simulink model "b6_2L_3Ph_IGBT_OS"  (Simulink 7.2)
settings: Solver=ode3  SolverMode=SingleTasking  StartTime=0.0  StopTime=0.1  FixedStep=10e-6  MaxStep=1e-5  RelTol=1e-4  AbsTol=1e-4
PreLoadFcn:
  | INIT_B6_2L_3Ph_IGBT_OS
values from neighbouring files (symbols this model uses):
  C = 10e-3*1    (= 0.01)    [INIT_B6_2L_3Ph_IGBT_OS.m]    (also in INIT_B6_3L_3Ph_IGBT_OS.m; INIT_MMC_100L.m = 0.005; INIT_MMC_200L.m = 0.005; INIT_MMC_20L.m)
  FS = 900    [INIT_B6_2L_3Ph_IGBT_OS.m]    (also in INIT_B6_3L_3Ph_IGBT_OS.m; INIT_PWM_2L.m = 1000; INIT_PWM_3L.m = 1000; INIT_PWM_Con.m = 1000)
  I_B = INS    [INIT_B6_2L_3Ph_IGBT_OS.m]    (also in INIT_B6_3L_3Ph_IGBT_OS.m; INIT_PWM_2L.m = INP; INIT_PWM_3L.m = INP; INIT_PWM_Con.m = INP)
  IDC = PDC/VDC    (= 166.666666667)    [INIT_B6_2L_3Ph_IGBT_OS.m]    (also in INIT_B6_3L_3Ph_IGBT_OS.m = 100; INIT_PWM_2L.m = 16.6666666667; INIT_PWM_3L.m = 83.3333333333; INIT_PWM_Con.m = 83.3333333333)
  LS = 1e-3    (= 0.001)    [INIT_B6_2L_3Ph_IGBT_OS.m]    (also in INIT_B6_3L_3Ph_IGBT_OS.m; INIT_MMC_100L.m = 0.025; INIT_MMC_200L.m = 0.025; INIT_MMC_20L.m = 0.0025)
  UC0 = 600    [INIT_B6_2L_3Ph_IGBT_OS.m]    (also in INIT_B6_3L_3Ph_IGBT_OS.m = 500; INIT_MMC_100L.m = 6800; INIT_MMC_200L.m = 3400; INIT_MMC_20L.m = 5000)
  UNS = ULLP/sqrt(3)    [INIT_B6_2L_3Ph_IGBT_OS.m]    (also in INIT_B6_3L_3Ph_IGBT_OS.m; INIT_MMC_100L.m = ULLP/sqrt(3)*340/400; INIT_MMC_200L.m = ULLP/sqrt(3)*340/400; INIT_MMC_20L.m)

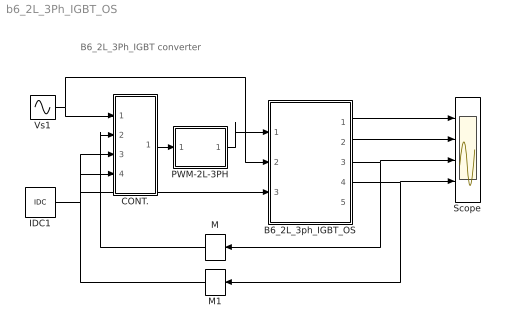
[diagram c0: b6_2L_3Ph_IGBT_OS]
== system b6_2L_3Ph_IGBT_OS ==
  note: B6_2L_3Ph_IGBT converter
  B6_2L_3ph_IGBT_OS : Subsystem  mask(B6 2-Level IGBT 3-Phase Converter){LS=LS, C=C, UC0=UC0, RL=1e6}
      mask prompts: LS "Source Inductance"; C "Load Cap"; UC0 "Initial Cap Voltage"; RL "Load Resistance"
      mask help: Input Vector u: u[0]= IGBT1.gate u[1]= IGBT2.gate u[2]= IGBT3.gate u[3]= IGBT4.gate u[4]= IGBT5.gate u[5]= IGBT6.gate u[6]= V1.V u[7]= V2.V u[8]= V3.V u[9]= IDC.i Output Vector y: y[0]= T1.I y[1]= D1.I y[2]= T1.V y[3]= T2.I y[4]= D2.I y[5]= T2.V y[6]= LS1.I y[7]= LS2.I y[8]= LS3.I y[9]= DC.V y[10]= Va.V y[11]= Vb.V y[12]= Vc.V Parameter Vector p: p[0]= Ls.L p[1]= C1.C p[2]= C1.vC0 p[3]= R1.r You can pause the simulation during running, change the Parameters you want and continue the Simulation
  CONT. : Subsystem
  IDC1 : Constant  Value=IDC
  M : Memory  Orientation=left
  M1 : Memory  Orientation=left
  PWM-2L-3PH : Subsystem  mask(PWM3-2L-3PH){FT=FS, PHT=0, DT=1e-6}
      mask prompts: FT "Triangular Frequency"; PHT "Trian. Phase Angle (Degree)"; DT "Dead Time"
      mask help: Pulse Width Modulation for 3 Phase Converter
  Scope : Scope  NumInputPorts=4
  Vs1 : Sin  Amplitude=UNS  Frequency=50*2*pi  Phase="[0  -2*pi/3   -4*pi/3]"  SampleTime=0
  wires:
  Vs1/1 -> CONT./1(UN), B6_2L_3ph_IGBT_OS/2(vS)
  IDC1/1 -> CONT./4(Id*), B6_2L_3ph_IGBT_OS/3(iDC)
  CONT./1(A) -> PWM-2L-3PH/1(In4)
  PWM-2L-3PH/1(Out1) -> B6_2L_3ph_IGBT_OS/1(SWs)
  B6_2L_3ph_IGBT_OS/3(iLs) -> Scope/3, M/1
  M/1 -> CONT./2(Iwr)
  B6_2L_3ph_IGBT_OS/1(iT1,iD1,vT1) -> Scope/1
  B6_2L_3ph_IGBT_OS/2(iT2,iD2,vT2) -> Scope/2
  B6_2L_3ph_IGBT_OS/4(vDC) -> Scope/4, M1/1
  M1/1 -> CONT./3(UDC)

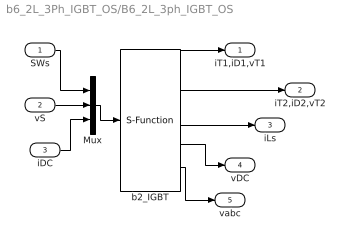
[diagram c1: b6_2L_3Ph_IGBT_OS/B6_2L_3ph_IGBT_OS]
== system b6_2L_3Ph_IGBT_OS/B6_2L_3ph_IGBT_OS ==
  SWs : Inport  OutDataType=sfix(16)  OutScaling=2^0
  vS : Inport  Port=2  OutDataType=sfix(16)  OutScaling=2^0
  iDC : Inport  Port=3  OutDataType=sfix(16)  OutScaling=2^0
  Mux : Mux  Inputs="[6  3  1]"
  b2_IGBT : S-Function  FunctionName=s_b6_2L_3Ph_IGBT_OS  Parameters="[ LS  C  UC0 RL]"  EnableBusSupport=off
  iT1,iD1,vT1 : Outport  OutDataType=sfix(16)  OutScaling=2^0
  iT2,iD2,vT2 : Outport  Port=2  OutDataType=sfix(16)  OutScaling=2^0
  iLs : Outport  Port=3  OutDataType=sfix(16)  OutScaling=2^0
  vDC : Outport  Port=4  OutDataType=sfix(16)  OutScaling=2^0
  vabc : Outport  Port=5  OutDataType=sfix(16)  OutScaling=2^0
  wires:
  b2_IGBT/5 -> vabc/1
  SWs/1 -> Mux/1
  vS/1 -> Mux/2
  b2_IGBT/1 -> iT1,iD1,vT1/1
  b2_IGBT/2 -> iT2,iD2,vT2/1
  b2_IGBT/3 -> iLs/1
  iDC/1 -> Mux/3
  Mux/1 -> b2_IGBT/1
  b2_IGBT/4 -> vDC/1

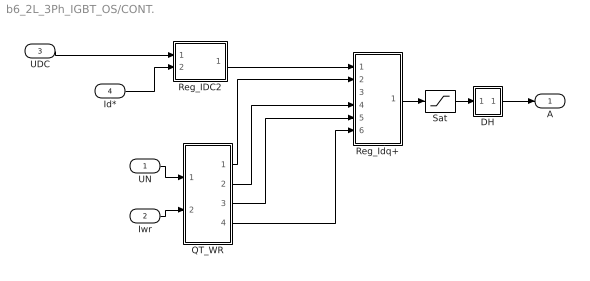
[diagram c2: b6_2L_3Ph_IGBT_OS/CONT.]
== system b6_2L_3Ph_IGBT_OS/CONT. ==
  UN : Inport
  Iwr : Inport  Port=2
  UDC : Inport  Port=3
  Id* : Inport  Port=4
  DH : Subsystem
  QT_WR : Subsystem
  Reg_IDC2 : Subsystem
  Reg_Idq+ : Subsystem
  Sat : Saturate  UpperLimit=1.5  LowerLimit=-1.5
  A : Outport
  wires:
  Sat/1 -> DH/1(I)
  Reg_Idq+/1(A+) -> Sat/1
  Id*/1 -> Reg_IDC2/2(Id*)
  DH/1(O) -> A/1
  UDC/1 -> Reg_IDC2/1(UDC)
  UN/1 -> QT_WR/1(UN)
  Iwr/1 -> QT_WR/2(I_WR)
  Reg_IDC2/1(Id1*) -> Reg_Idq+/1(Id1*)
  QT_WR/3(th1) -> Reg_Idq+/5(th)
  QT_WR/2(Iq1) -> Reg_Idq+/4(Iq1)
  QT_WR/1(Id1) -> Reg_Idq+/2(Id1)
  QT_WR/4(Ud) -> Reg_Idq+/6(Ud)

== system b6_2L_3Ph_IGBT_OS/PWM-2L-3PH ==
  In4 : Inport  OutDataType=sfix(16)  OutScaling=2^0
  Demux : Demux  Outputs=3
  Mux : Mux  Inputs=3
  PWM-2L-1PH : Subsystem  mask(PWM-2L-1PH){FT=FT, PHT=PHT, DT=DT}
      mask prompts: FT "Triangular Frequency"; PHT "Trian. Phase Angle (Degree)"; DT "Dead Time"
      mask help: Pulse Width Modulation for 1 Phase Converter
  PWM-2L-1PH1 : Subsystem  mask(PWM-2L-1PH){FT=FT, PHT=PHT, DT=DT}
      mask prompts: FT "Triangular Frequency"; PHT "Trian. Phase Angle (Degree)"; DT "Dead Time"
      mask help: Pulse Width Modulation for 1 Phase Converter
  PWM-2L-1PH2 : Subsystem  mask(PWM-2L-1PH){FT=FT, PHT=PHT, DT=DT}
      mask prompts: FT "Triangular Frequency"; PHT "Trian. Phase Angle (Degree)"; DT "Dead Time"
      mask help: Pulse Width Modulation for 1 Phase Converter
  Out1 : Outport
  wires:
  In4/1 -> Demux/1
  Demux/3 -> PWM-2L-1PH2/1(In1)
  Demux/2 -> PWM-2L-1PH1/1(In1)
  Demux/1 -> PWM-2L-1PH/1(In1)
  PWM-2L-1PH1/1(Out1) -> Mux/2
  PWM-2L-1PH/1(Out1) -> Mux/1
  PWM-2L-1PH2/1(Out1) -> Mux/3
  Mux/1 -> Out1/1

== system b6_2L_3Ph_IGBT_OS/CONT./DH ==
  I : Inport
  Gain : Gain  Gain=0.5
  MinMax : MinMax
  MinMax1 : MinMax  Function=max
  Sum6 : Sum  Inputs=--
  Sum7 : Sum
  O : Outport  InitialOutput=0
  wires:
  I/1 -> MinMax1/1, MinMax/1, Sum7/1
  MinMax/1 -> Sum6/1
  MinMax1/1 -> Sum6/2
  Sum6/1 -> Gain/1
  Gain/1 -> Sum7/2
  Sum7/1 -> O/1

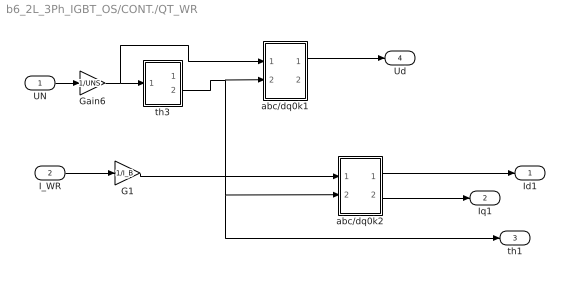
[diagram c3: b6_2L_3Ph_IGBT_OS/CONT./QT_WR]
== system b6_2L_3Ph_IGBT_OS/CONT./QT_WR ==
  UN : Inport
  I_WR : Inport  Port=2
  G1 : Gain  Gain=1/I_B
  Gain6 : Gain  Gain=1/UNS
  abc/dq0k1 : Subsystem
  abc/dq0k2 : Subsystem
  th3 : Subsystem
  Id1 : Outport
  Iq1 : Outport  Port=2
  th1 : Outport  Port=3
  Ud : Outport  Port=4
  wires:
  th3/2(th) -> abc/dq0k2/2(th), th1/1, abc/dq0k1/2(th)
  I_WR/1 -> G1/1
  G1/1 -> abc/dq0k2/1(a)
  UN/1 -> Gain6/1
  Gain6/1 -> th3/1(abc), abc/dq0k1/1(a)
  abc/dq0k2/1(dk) -> Id1/1
  abc/dq0k2/2(qk) -> Iq1/1
  abc/dq0k1/1(dk) -> Ud/1

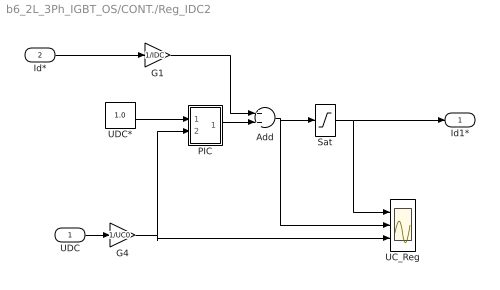
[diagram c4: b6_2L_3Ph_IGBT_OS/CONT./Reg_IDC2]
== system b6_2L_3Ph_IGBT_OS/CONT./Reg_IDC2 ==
  UDC : Inport
  Id* : Inport  Port=2
  Add : Sum
  G1 : Gain  Gain=1/IDC
  G4 : Gain  Gain=1/UC0
  PIC : Subsystem  mask(PI-controller){Kp=1, Ki=10, lim=2, Ts=-1}
      mask prompts: Kp "Proportional gain (Kp)"; Ki "Integral gain (Ki)"; lim "Output limit"; Ts "Sampling time (s)"
      mask help: Proportional-Integral Controller
  Sat : Saturate  UpperLimit=2  LowerLimit=-2
  UC_Reg : Scope  NumInputPorts=3
  UDC* : Constant  Value=1.0
  Id1* : Outport
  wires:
  Id*/1 -> G1/1
  PIC/1(e*) -> Add/2
  Sat/1 -> Id1*/1, UC_Reg/1
  Add/1 -> Sat/1, UC_Reg/2
  G4/1 -> UC_Reg/3, PIC/2(c)
  UDC*/1 -> PIC/1(c*)
  UDC/1 -> G4/1
  G1/1 -> Add/1

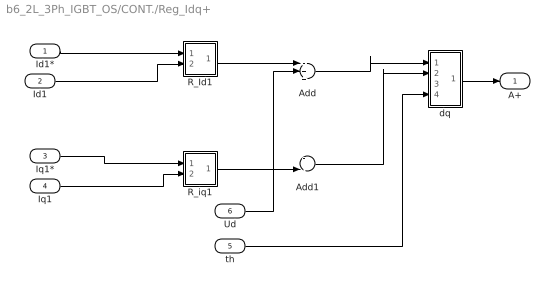
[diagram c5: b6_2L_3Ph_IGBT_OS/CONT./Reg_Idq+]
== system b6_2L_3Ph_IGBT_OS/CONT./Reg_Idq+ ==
  Id1* : Inport
  Id1 : Inport  Port=2
  Iq1* : Inport  Port=3
  Iq1 : Inport  Port=4
  th : Inport  Port=5
  Ud : Inport  Port=6
  Add : Sum  Inputs=-++
  Add1 : Sum  Inputs=--
  R_Id1 : Subsystem  mask(PI-controller){Kp=0.1, Ki=200, lim=2, Ts=-1}
      mask prompts: Kp "Proportional gain (Kp)"; Ki "Integral gain (Ki)"; lim "Output limit"; Ts "Sampling time (s)"
      mask help: Proportional-Integral Controller
  R_iq1 : Subsystem  mask(PI-controller){Kp=0.1, Ki=200, lim=2, Ts=-2}
      mask prompts: Kp "Proportional gain (Kp)"; Ki "Integral gain (Ki)"; lim "Output limit"; Ts "Sampling time (s)"
      mask help: Proportional-Integral Controller
  dq : Subsystem
  A+ : Outport
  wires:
  Iq1/1 -> R_iq1/2(c)
  Iq1*/1 -> R_iq1/1(c*)
  Id1/1 -> R_Id1/2(c)
  Id1*/1 -> R_Id1/1(c*)
  dq/1(a) -> A+/1
  th/1 -> dq/4(th)
  R_Id1/1(e*) -> Add/1
  R_iq1/1(e*) -> Add1/2
  Add/1 -> dq/1(dk)
  Add1/1 -> dq/2(qk)
  Ud/1 -> Add/2

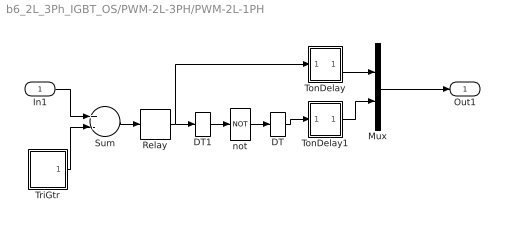
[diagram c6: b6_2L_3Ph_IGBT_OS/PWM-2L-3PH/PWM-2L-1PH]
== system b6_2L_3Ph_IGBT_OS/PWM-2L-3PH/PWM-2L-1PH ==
  In1 : Inport  OutDataType=sfix(16)  OutScaling=2^0
  DT : DataTypeConversion
  DT1 : DataTypeConversion
  Mux : Mux  Inputs=2
  Relay : Relay  OutDataType=sfix(16)  OutScaling=2^0
  Sum : Sum  Inputs=+-  OutDataType=sfix(16)  OutScaling=2^0
  TonDelay : Subsystem  mask(TonDelay){DT=DT}
      mask prompts: DT "Dead Time"
      mask help: Turn on dead time to protect against short circuit of the converter leg
  TonDelay1 : Subsystem  mask(TonDelay){DT=DT}
      mask prompts: DT "Dead Time"
      mask help: Turn on dead time to protect against short circuit of the converter leg
  TriGtr : Subsystem  mask(TriGtr){T=1/FT, Td=PHT/FT/360}
      mask prompts: T "Period Time"; Td "Time Delay"
      mask help: Triangular Wave Generator with variable time delay
  not : Logic  Operator=NOT  Inputs=1
  Out1 : Outport  InitialOutput=0
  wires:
  Mux/1 -> Out1/1
  TonDelay/1(s1d) -> Mux/1
  Relay/1 -> TonDelay/1(s1), DT1/1
  TonDelay1/1(s1d) -> Mux/2
  not/1 -> DT/1
  Sum/1 -> Relay/1
  TriGtr/1(O) -> Sum/2
  In1/1 -> Sum/1
  DT/1 -> TonDelay1/1(s1)
  DT1/1 -> not/1

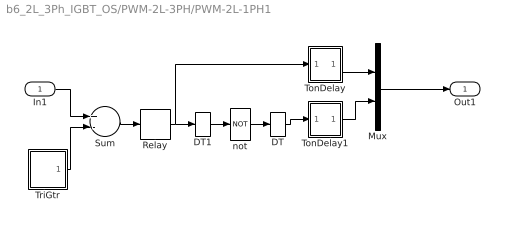
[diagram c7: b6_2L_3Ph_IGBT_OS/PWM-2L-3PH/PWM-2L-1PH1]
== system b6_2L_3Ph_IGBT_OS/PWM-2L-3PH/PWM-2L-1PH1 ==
  In1 : Inport  OutDataType=sfix(16)  OutScaling=2^0
  DT : DataTypeConversion
  DT1 : DataTypeConversion
  Mux : Mux  Inputs=2
  Relay : Relay  OutDataType=sfix(16)  OutScaling=2^0
  Sum : Sum  Inputs=+-  OutDataType=sfix(16)  OutScaling=2^0
  TonDelay : Subsystem  mask(TonDelay){DT=DT}
      mask prompts: DT "Dead Time"
      mask help: Turn on dead time to protect against short circuit of the converter leg
  TonDelay1 : Subsystem  mask(TonDelay){DT=DT}
      mask prompts: DT "Dead Time"
      mask help: Turn on dead time to protect against short circuit of the converter leg
  TriGtr : Subsystem  mask(TriGtr){T=1/FT, Td=PHT/FT/360}
      mask prompts: T "Period Time"; Td "Time Delay"
      mask help: Triangular Wave Generator with variable time delay
  not : Logic  Operator=NOT  Inputs=1
  Out1 : Outport  InitialOutput=0
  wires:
  DT1/1 -> not/1
  DT/1 -> TonDelay1/1(s1)
  In1/1 -> Sum/1
  TriGtr/1(O) -> Sum/2
  Sum/1 -> Relay/1
  not/1 -> DT/1
  TonDelay1/1(s1d) -> Mux/2
  Relay/1 -> DT1/1, TonDelay/1(s1)
  TonDelay/1(s1d) -> Mux/1
  Mux/1 -> Out1/1

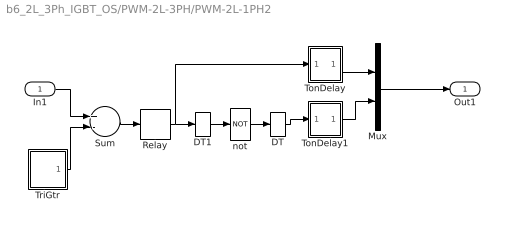
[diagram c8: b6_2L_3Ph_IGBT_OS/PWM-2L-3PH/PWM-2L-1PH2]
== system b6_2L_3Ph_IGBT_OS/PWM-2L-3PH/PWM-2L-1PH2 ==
  In1 : Inport  OutDataType=sfix(16)  OutScaling=2^0
  DT : DataTypeConversion
  DT1 : DataTypeConversion
  Mux : Mux  Inputs=2
  Relay : Relay  OutDataType=sfix(16)  OutScaling=2^0
  Sum : Sum  Inputs=+-  OutDataType=sfix(16)  OutScaling=2^0
  TonDelay : Subsystem  mask(TonDelay){DT=DT}
      mask prompts: DT "Dead Time"
      mask help: Turn on dead time to protect against short circuit of the converter leg
  TonDelay1 : Subsystem  mask(TonDelay){DT=DT}
      mask prompts: DT "Dead Time"
      mask help: Turn on dead time to protect against short circuit of the converter leg
  TriGtr : Subsystem  mask(TriGtr){T=1/FT, Td=PHT/FT/360}
      mask prompts: T "Period Time"; Td "Time Delay"
      mask help: Triangular Wave Generator with variable time delay
  not : Logic  Operator=NOT  Inputs=1
  Out1 : Outport  InitialOutput=0
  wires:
  Mux/1 -> Out1/1
  TonDelay/1(s1d) -> Mux/1
  Relay/1 -> TonDelay/1(s1), DT1/1
  TonDelay1/1(s1d) -> Mux/2
  not/1 -> DT/1
  Sum/1 -> Relay/1
  TriGtr/1(O) -> Sum/2
  In1/1 -> Sum/1
  DT/1 -> TonDelay1/1(s1)
  DT1/1 -> not/1

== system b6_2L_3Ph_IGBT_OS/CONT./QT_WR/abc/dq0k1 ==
  a : Inport
  th : Inport  Port=2
  Demux : Demux  Outputs=3
  Fcn : Fcn  Expr=u(1)*cos(u(3)) + u(2)*sin(u(3))
  Fcn1 : Fcn  Expr=-u(1)*sin(u(3)) + u(2)*cos(u(3))
  K : Gain  Gain="2/3*[1   -.5   -.5;  0   sqrt(3)/2   -sqrt(3)/2;  .5    .5    .5]"  Multiplication=Matrix(K*u)
  Mux1 : Mux  Inputs=3
  dk : Outport
  qk : Outport  Port=2
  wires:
  Demux/2 -> Mux1/2
  Demux/1 -> Mux1/1
  th/1 -> Mux1/3
  Fcn1/1 -> qk/1
  Fcn/1 -> dk/1
  Mux1/1 -> Fcn/1, Fcn1/1
  a/1 -> K/1
  K/1 -> Demux/1

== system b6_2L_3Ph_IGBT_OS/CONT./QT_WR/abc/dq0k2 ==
  a : Inport
  th : Inport  Port=2
  Demux : Demux  Outputs=3
  Fcn : Fcn  Expr=u(1)*cos(u(3)) + u(2)*sin(u(3))
  Fcn1 : Fcn  Expr=-u(1)*sin(u(3)) + u(2)*cos(u(3))
  K : Gain  Gain="2/3*[1   -.5   -.5;  0   sqrt(3)/2   -sqrt(3)/2;  .5    .5    .5]"  Multiplication=Matrix(K*u)
  Mux1 : Mux  Inputs=3
  dk : Outport
  qk : Outport  Port=2
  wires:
  K/1 -> Demux/1
  a/1 -> K/1
  Mux1/1 -> Fcn1/1, Fcn/1
  Fcn/1 -> dk/1
  Fcn1/1 -> qk/1
  th/1 -> Mux1/3
  Demux/1 -> Mux1/1
  Demux/2 -> Mux1/2

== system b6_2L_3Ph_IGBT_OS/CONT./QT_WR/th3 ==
  abc : Inport
  C : ComplexToMagnitudeAngle
  Demux : Demux  Outputs=3
  K : Gain  Gain="2/3*[1   -.5   -.5;  0   sqrt(3)/2   -sqrt(3)/2;  .5    .5    .5]"  Multiplication=Matrix(K*u)
  R : RealImagToComplex
  |u| : Outport
  th : Outport  Port=2
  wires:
  C/2 -> th/1
  R/1 -> C/1
  Demux/2 -> R/2
  Demux/1 -> R/1
  abc/1 -> K/1
  K/1 -> Demux/1
  C/1 -> |u|/1

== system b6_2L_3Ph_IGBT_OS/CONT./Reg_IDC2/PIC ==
  c* : Inport  OutDataType=sfix(16)  OutScaling=2^0
  c : Inport  Port=2  OutDataType=sfix(16)  OutScaling=2^0
  Gain : Gain  Gain=Ki  ParameterDataType=sfix(16)  ParameterScaling=2^0  OutDataType=sfix(16)  OutScaling=2^0
  Gain1 : Gain  Gain=Kp  ParameterDataType=sfix(16)  ParameterScaling=2^0  OutDataType=sfix(16)  OutScaling=2^0
  Integrator : Integrator  UpperSaturationLimit=lim  LowerSaturationLimit=-lim
  Saturation : Saturate  UpperLimit=lim  LowerLimit=-lim
  Sum1 : Sum  Inputs=+-  OutDataType=sfix(16)  OutScaling=2^0
  Sum2 : Sum  OutDataType=sfix(16)  OutScaling=2^0
  e* : Outport  InitialOutput=0
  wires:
  Integrator/1 -> Sum2/2
  c*/1 -> Sum1/1
  c/1 -> Sum1/2
  Saturation/1 -> e*/1
  Sum2/1 -> Saturation/1
  Sum1/1 -> Gain1/1, Gain/1
  Gain1/1 -> Sum2/1
  Gain/1 -> Integrator/1

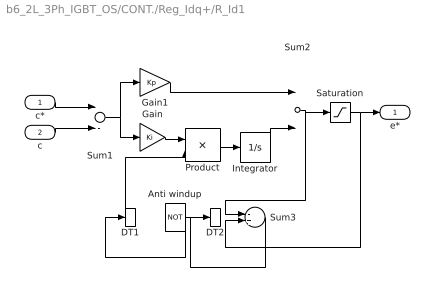
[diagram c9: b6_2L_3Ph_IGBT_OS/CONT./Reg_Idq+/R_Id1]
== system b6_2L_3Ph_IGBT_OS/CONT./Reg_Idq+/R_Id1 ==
  c* : Inport
  c : Inport  Port=2
  Anti windup : Logic  Operator=NOT
  DT1 : DataTypeConversion
  DT2 : DataTypeConversion
  Gain : Gain  Gain=Ki
  Gain1 : Gain  Gain=Kp
  Integrator : Integrator  UpperSaturationLimit=lim  LowerSaturationLimit=-lim
  Product : Product
  Saturation : Saturate  UpperLimit=lim  LowerLimit=-lim
  Sum1 : Sum  Inputs=+-
  Sum2 : Sum
  Sum3 : Sum  Inputs=-+
  e* : Outport  InitialOutput=0
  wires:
  Integrator/1 -> Sum2/2
  c*/1 -> Sum1/1
  c/1 -> Sum1/2
  Saturation/1 -> e*/1, Sum3/2
  Sum2/1 -> Saturation/1, Sum3/1
  Sum1/1 -> Gain1/1, Gain/1
  Gain1/1 -> Sum2/1
  Anti windup/1 -> DT1/1
  DT1/1 -> Product/2
  Gain/1 -> Product/1
  Product/1 -> Integrator/1
  DT2/1 -> Anti windup/1
  Sum3/1 -> DT2/1

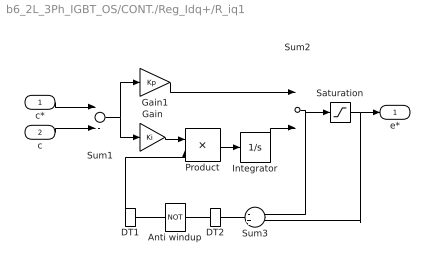
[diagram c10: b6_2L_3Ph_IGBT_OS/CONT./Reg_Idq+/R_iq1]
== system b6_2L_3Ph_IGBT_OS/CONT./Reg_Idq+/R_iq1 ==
  c* : Inport
  c : Inport  Port=2
  Anti windup : Logic  Operator=NOT
  DT1 : DataTypeConversion
  DT2 : DataTypeConversion
  Gain : Gain  Gain=Ki
  Gain1 : Gain  Gain=Kp
  Integrator : Integrator  UpperSaturationLimit=lim  LowerSaturationLimit=-lim
  Product : Product
  Saturation : Saturate  UpperLimit=lim  LowerLimit=-lim
  Sum1 : Sum  Inputs=+-
  Sum2 : Sum
  Sum3 : Sum  Inputs=-+
  e* : Outport  InitialOutput=0
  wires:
  Sum3/1 -> DT2/1
  DT2/1 -> Anti windup/1
  Product/1 -> Integrator/1
  Gain/1 -> Product/1
  DT1/1 -> Product/2
  Anti windup/1 -> DT1/1
  Gain1/1 -> Sum2/1
  Sum1/1 -> Gain/1, Gain1/1
  Sum2/1 -> Sum3/1, Saturation/1
  Saturation/1 -> Sum3/2, e*/1
  c/1 -> Sum1/2
  c*/1 -> Sum1/1
  Integrator/1 -> Sum2/2

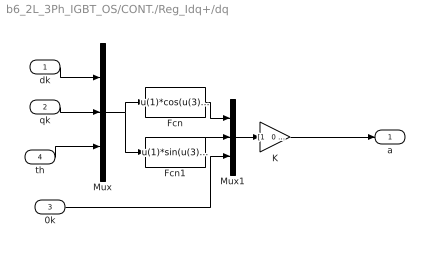
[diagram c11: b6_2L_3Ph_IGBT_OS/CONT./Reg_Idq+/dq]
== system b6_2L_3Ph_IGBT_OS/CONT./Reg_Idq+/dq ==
  dk : Inport
  qk : Inport  Port=2
  0k : Inport  Port=3
  th : Inport  Port=4
  Fcn : Fcn  Expr=u(1)*cos(u(3)) - u(2)*sin(u(3))
  Fcn1 : Fcn  Expr=u(1)*sin(u(3)) + u(2)*cos(u(3))
  K : Gain  Gain="[1   0  1 ;  -.5   sqrt(3)/2    1 ;  -.5    -sqrt(3)/2    1]"  Multiplication=Matrix(K*u)
  Mux : Mux  Inputs=3
  Mux1 : Mux  Inputs=3
  a : Outport
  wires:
  0k/1 -> Mux1/3
  th/1 -> Mux/3
  Fcn1/1 -> Mux1/2
  Fcn/1 -> Mux1/1
  Mux1/1 -> K/1
  K/1 -> a/1
  Mux/1 -> Fcn1/1, Fcn/1
  qk/1 -> Mux/2
  dk/1 -> Mux/1

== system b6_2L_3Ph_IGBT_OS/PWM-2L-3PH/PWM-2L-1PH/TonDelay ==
  s1 : Inport  Orientation=down  OutDataType=sfix(16)  OutScaling=2^0
  Int : Integrator  ExternalReset=falling
  Rel1 : Relay  OnSwitchValue=DT  OutDataType=sfix(16)  OutScaling=2^0
  s1d : Outport  InitialOutput=0
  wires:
  Rel1/1 -> s1d/1
  s1/1 -> Int/1, Int/2
  Int/1 -> Rel1/1

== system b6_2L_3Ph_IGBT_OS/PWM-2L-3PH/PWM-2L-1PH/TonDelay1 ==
  s1 : Inport  Orientation=down  OutDataType=sfix(16)  OutScaling=2^0
  Int : Integrator  ExternalReset=falling
  Rel1 : Relay  OnSwitchValue=DT  OutDataType=sfix(16)  OutScaling=2^0
  s1d : Outport  InitialOutput=0
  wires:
  Rel1/1 -> s1d/1
  s1/1 -> Int/1, Int/2
  Int/1 -> Rel1/1

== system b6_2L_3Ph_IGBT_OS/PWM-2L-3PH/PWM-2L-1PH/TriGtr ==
  Clock : Clock
  S2 : Subsystem
  Sum : Sum  OutDataType=sfix(16)  OutScaling=2^0
  T : Constant  Value=T  OutDataType=sfix(16)  OutScaling=2^0
  Td : Constant  Value=Td  OutDataType=sfix(16)  OutScaling=2^0
  mod : Math  Operator=mod
  O : Outport  InitialOutput=0
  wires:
  Td/1 -> Sum/2
  Sum/1 -> mod/1
  T/1 -> mod/2
  Clock/1 -> Sum/1
  S2/1(O1) -> O/1
  mod/1 -> S2/1(I1)

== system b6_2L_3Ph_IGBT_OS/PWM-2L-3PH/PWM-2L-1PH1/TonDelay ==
  s1 : Inport  Orientation=down  OutDataType=sfix(16)  OutScaling=2^0
  Int : Integrator  ExternalReset=falling
  Rel1 : Relay  OnSwitchValue=DT  OutDataType=sfix(16)  OutScaling=2^0
  s1d : Outport  InitialOutput=0
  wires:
  Int/1 -> Rel1/1
  s1/1 -> Int/2, Int/1
  Rel1/1 -> s1d/1

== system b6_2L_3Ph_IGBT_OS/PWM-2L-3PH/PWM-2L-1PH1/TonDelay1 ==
  s1 : Inport  Orientation=down  OutDataType=sfix(16)  OutScaling=2^0
  Int : Integrator  ExternalReset=falling
  Rel1 : Relay  OnSwitchValue=DT  OutDataType=sfix(16)  OutScaling=2^0
  s1d : Outport  InitialOutput=0
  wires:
  Int/1 -> Rel1/1
  s1/1 -> Int/2, Int/1
  Rel1/1 -> s1d/1

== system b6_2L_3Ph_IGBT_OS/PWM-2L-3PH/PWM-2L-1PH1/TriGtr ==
  Clock : Clock
  S2 : Subsystem
  Sum : Sum  OutDataType=sfix(16)  OutScaling=2^0
  T : Constant  Value=T  OutDataType=sfix(16)  OutScaling=2^0
  Td : Constant  Value=Td  OutDataType=sfix(16)  OutScaling=2^0
  mod : Math  Operator=mod
  O : Outport  InitialOutput=0
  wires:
  mod/1 -> S2/1(I1)
  S2/1(O1) -> O/1
  Clock/1 -> Sum/1
  T/1 -> mod/2
  Sum/1 -> mod/1
  Td/1 -> Sum/2

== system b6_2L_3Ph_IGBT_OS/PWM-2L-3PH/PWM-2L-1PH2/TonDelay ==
  s1 : Inport  Orientation=down  OutDataType=sfix(16)  OutScaling=2^0
  Int : Integrator  ExternalReset=falling
  Rel1 : Relay  OnSwitchValue=DT  OutDataType=sfix(16)  OutScaling=2^0
  s1d : Outport  InitialOutput=0
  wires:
  Rel1/1 -> s1d/1
  s1/1 -> Int/1, Int/2
  Int/1 -> Rel1/1

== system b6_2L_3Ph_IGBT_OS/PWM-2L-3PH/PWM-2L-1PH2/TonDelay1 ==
  s1 : Inport  Orientation=down  OutDataType=sfix(16)  OutScaling=2^0
  Int : Integrator  ExternalReset=falling
  Rel1 : Relay  OnSwitchValue=DT  OutDataType=sfix(16)  OutScaling=2^0
  s1d : Outport  InitialOutput=0
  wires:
  Rel1/1 -> s1d/1
  s1/1 -> Int/1, Int/2
  Int/1 -> Rel1/1

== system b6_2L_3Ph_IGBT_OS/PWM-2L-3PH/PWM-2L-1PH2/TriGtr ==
  Clock : Clock
  S2 : Subsystem
  Sum : Sum  OutDataType=sfix(16)  OutScaling=2^0
  T : Constant  Value=T  OutDataType=sfix(16)  OutScaling=2^0
  Td : Constant  Value=Td  OutDataType=sfix(16)  OutScaling=2^0
  mod : Math  Operator=mod
  O : Outport  InitialOutput=0
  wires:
  Td/1 -> Sum/2
  Sum/1 -> mod/1
  T/1 -> mod/2
  Clock/1 -> Sum/1
  S2/1(O1) -> O/1
  mod/1 -> S2/1(I1)

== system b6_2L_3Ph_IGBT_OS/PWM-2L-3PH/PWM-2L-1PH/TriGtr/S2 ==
  I1 : Inport
  Fcn : Fcn  Expr="(u* (u <=T/4) * 4/T)   +  (  (u > T/4) && ( u <=3*T/4) )* ( 1 - (u-T/4) *4/T )   +  ( (u > 3*T/4)&& (u<=T)) * ( ((u -3*T/4)* 4/T )-1 )"
  O1 : Outport
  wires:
  I1/1 -> Fcn/1
  Fcn/1 -> O1/1

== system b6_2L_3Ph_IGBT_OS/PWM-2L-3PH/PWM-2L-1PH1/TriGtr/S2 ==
  I1 : Inport
  Fcn : Fcn  Expr="(u* (u <=T/4) * 4/T)   +  (  (u > T/4) && ( u <=3*T/4) )* ( 1 - (u-T/4) *4/T )   +  ( (u > 3*T/4)&& (u<=T)) * ( ((u -3*T/4)* 4/T )-1 )"
  O1 : Outport
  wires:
  Fcn/1 -> O1/1
  I1/1 -> Fcn/1

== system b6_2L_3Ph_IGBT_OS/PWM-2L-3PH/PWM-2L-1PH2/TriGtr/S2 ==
  I1 : Inport
  Fcn : Fcn  Expr="(u* (u <=T/4) * 4/T)   +  (  (u > T/4) && ( u <=3*T/4) )* ( 1 - (u-T/4) *4/T )   +  ( (u > 3*T/4)&& (u<=T)) * ( ((u -3*T/4)* 4/T )-1 )"
  O1 : Outport
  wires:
  I1/1 -> Fcn/1
  Fcn/1 -> O1/1
